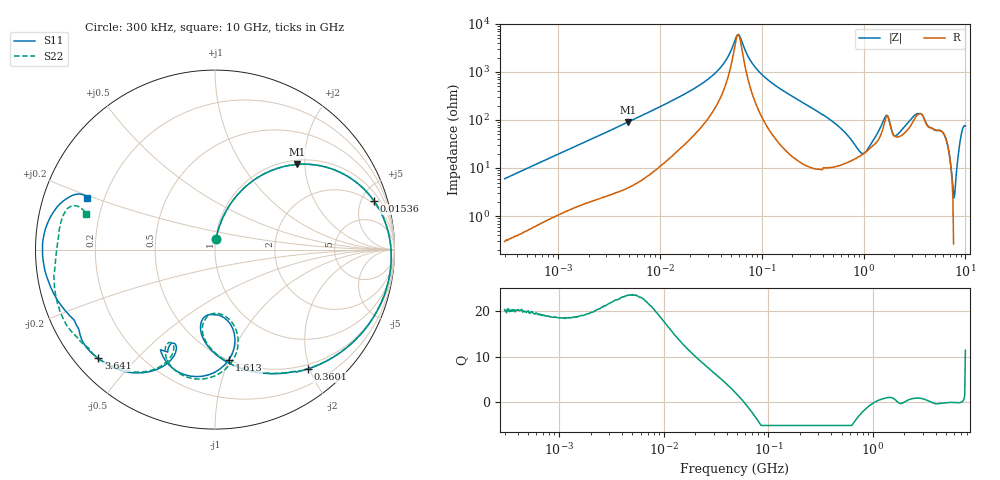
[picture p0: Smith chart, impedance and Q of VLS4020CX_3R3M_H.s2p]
! S-Parameter Data Generated by TDK Corporation
! Copyright(C) 2024 TDK Corporation.
! All Rights Reserved.
! TDK P/N: VLS4020CX-3R3M-H (SMD / SMT Inductor (Coil))
! Property: L=3.3uH at 1MHz
! Size(LxWxT): 4x4x2mm
! Model Type: s2p (Touchstone File Format Version 1.0)
! Frequency: DC=Yes Start=0.3MHz Stop=10000MHz 802points Log-sweep
! Model Generated on May 28, 2024
! Terms and conditions regarding TDK Simulation Models:
! 1)This simulation model is being provided solely for informational
!  purposes. Please refer to the specifications of the products in
!  terms of detailed characteristics of such products.
! 2)In no event shall TDK Corporation of any of its subsidiaries be
!  liable for any loss or damage arising, directly or indirectly,
!  from any information contained in this simulation model, including,
!  but not limited to loss or damages arising from any inaccuracies,
!  omissions or errors in connection with such information.
! 3)Any and all copyrights on this simulation model are owned by
!  TDK Corporation.  Duplication or redistribution of this simulation
!  model without prior written permission from TDK Corporation
!  is prohibited.
! 4)This simulation model is subject to any modification or change
!  without any prior notice.
! 5)Neither TDK Corporation nor any of its subsidiaries shall make any
!  warranty, express or implied, including but not limited to the
!  correctness, implied warranties of merchantability and fitness for
!  a particular purpose with respect to this simulation models.
! 6)The use of this simulation model shall be deemed to have consented
!  to the terms and conditions hereof.
! Port Assignments:
!  1 ---@@@--- 2
! Applicable Conditions:
!  Temperature = 25 degC
!  DC Bias Current = 0 A
!  Small Signal Operation
# Hz S MA R 50
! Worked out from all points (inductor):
!   801 points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, 300 kHz to 10 GHz, reference 50 ohm
!   read as one part in series: L = 3.15 uH near 318.3 kHz
!   highest Q = 23.4 at 4.921 MHz (marker M1), where L = 2.95 uH
!   self-resonance near 58.03 MHz
!   S11 on the Smith chart (normalised r, x): 300 kHz: 1.01, +0.12; 15.36 MHz: 1.64, +6.25; 360.1 MHz: 0.43, -1.98; 1.613 GHz: 0.50, -1.00; 3.641 GHz: 0.07, -0.39; 10 GHz: 0.13, +0.19
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300000  0.05924 83.6  0.9954 -3.5  0.9952 -3.4  0.05922 83.8
1713600  0.3032 69.2  0.9371 -17.7  0.937 -17.7  0.3031 69.2
4920797  0.659 46.1  0.7245 -41.5  0.7244 -41.5  0.6589 46.1
9671944  0.8558 27.5  0.472 -59.3  0.472 -59.3  0.8558 27.5
1.535588e7  0.9262 17.1  0.3107 -68.4  0.3107 -68.4  0.9262 17.1
3.642588e7  0.9762 3.0  0.09507 -75.2  0.09508 -75.2  0.9762 3.1
5.477226e7  0.9832 -2.7  0.02137 -41.6  0.02137 -41.6  0.9832 -2.7
6.057755e7  0.9838 -4.2  0.0171 15.8  0.0171 15.8  0.9838 -4.1
7.683413e7  0.9835 -7.9  0.0544 66.2  0.05439 66.2  0.9835 -7.8
1.063884e8  0.9786 -13.7  0.122 69.8  0.122 69.8  0.9784 -13.6
3.126428e8  0.8749 -45.8  0.4382 41.5  0.4382 41.5  0.8752 -45.5
3.601167e8  0.8434 -52.0  0.4881 35.1  0.4881 35.1  0.844 -51.5
8.643532e8  0.5304 -95.0  0.7097 -19.4  0.7098 -19.4  0.536 -93.8
1.323741e9  0.3648 -87.5  0.6476 -63.4  0.6477 -63.4  0.3546 -89.7
1.613252e9  0.6195 -82.9  0.3705 -89.6  0.371 -89.6  0.6186 -80.3
1.767019e9  0.7179 -100.8  0.2928 -68.8  0.2931 -68.9  0.7281 -97.8
1.942751e9  0.6599 -116.2  0.3965 -67.6  0.3968 -67.7  0.6808 -112.5
2.38587e9  0.584 -111.6  0.4037 -103.7  0.4042 -103.8  0.5876 -113.0
3.640519e9  0.8891 -137.0  0.09764 -121.7  0.09715 -121.9  0.8779 -133.5
5.849356e9  0.8955 -156.9  0.07992 -130.5  0.07988 -130.5  0.927 -152.6
7.540283e9  0.9611 -178.1  0.05813 -132.1  0.05795 -132.3  0.8919 -175.5
1e10  0.7713 158.0  0.04605 -127.4  0.0463 -127.1  0.7459 164.4
